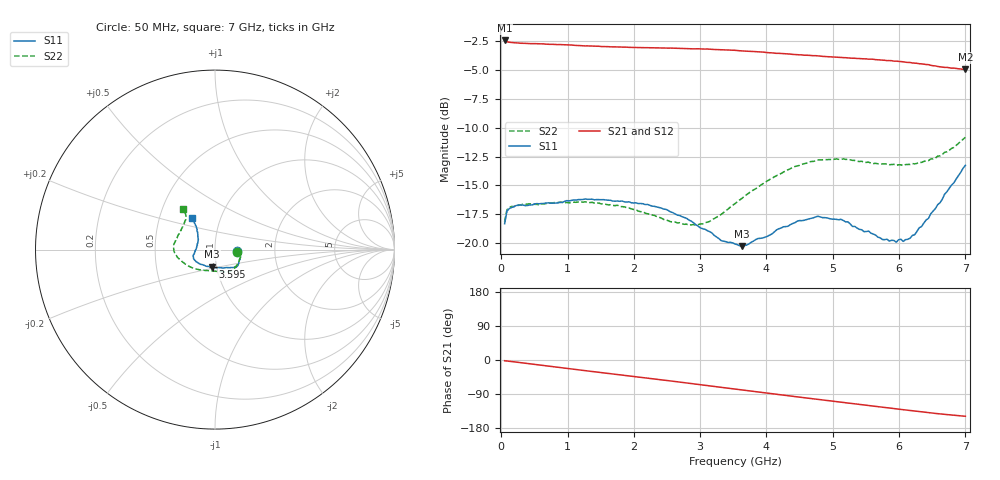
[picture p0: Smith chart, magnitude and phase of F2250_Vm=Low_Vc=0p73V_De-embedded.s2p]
! Integrated Device Technology
! Corporate Headquarters
! 6024 Silver Creek Valley Road
! San Jose, CA 95138  USA
! Phone:  1-408-284-8200
! Toll Free:  1-800-223-1366
! Webpage:  http://www.idt.com/
! Timing and RF Division
! 515 Groton Road, Suite 102
! Westford, MA 01886-6024
! Device:  F2250
! Description: Voltage Variable RF Attenuator
! Frequency:  50.0 -  6000.00 MHz
! Package:  3x3 mm Thin QFN Plastic Package: 16 pin
! Ports:  2 RF, 3 DC
!  Pin  1  = GND
!  Pin  2  = NC
!  Pin  3  = RF1  = Port 1
!  Pin  4  = NC
!  Pin  5  = GND
!  Pin  6  = GND
!  Pin  7  = GND
!  Pin  8  = GND
!  Pin  9  = NC
!  Pin 10  = RF2  = Port 2
!  Pin 11  = NC
!  Pin 12  = GND
!  Pin 13  = GND
!  Pin 14  = VCNTRL
!  Pin 15  = VDD
!  Pin 16  = VMODE
! Vcntrl:  0.730 Volts
! Vmode:  +0.000 Volts
! Vdd:  +3.30  Volts
! Current:  1.156 mA
! Data:  The device was measured on a the F2250 evaluation board which has
!  individual transmission lines to the RF pins.  Data was collected
!  using a calibrated network analyzer.  The evaluation board was
!  de-embedded using a TRL calibration technique.
!  The reference plane is the edge of the package pin.
! Misc:  SN 10
!  Action Tracker AT0258
! Date Measured:  2014-11-26
! Date:  2015-10-15  MJV
! Note:
!  Integrated Device Technology supplies this data as a sample of measured
!  data at the package pin for this product.  Your particular data for this
!  product may vary.
!  Data was taken at 25 degrees C.
!  Integrated Device Technology reserves the right to change this data at anytime.
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# GHz S dB R 50
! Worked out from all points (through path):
!   201 points, 50 MHz to 7 GHz, reference 50 ohm
!   highest |S21| = -2.45 dB at 50 MHz (marker M1); lowest = -5.0 dB at 7 GHz (marker M2)
!   group delay of S21, straight-line fit = 59.6 ps
!   lowest |S11| = -20.3 dB at 3.629 GHz (marker M3), VSWR 1.21, Z = 47.5 - j9.18 ohm
!   |S11| at or under -10 dB: start of sweep to end of sweep
!   |S22| runs from -18.4 to -10.8 dB; largest |S21 - S12| = 0.0014
!   S11 on the Smith chart (normalised r, x): 50 MHz: 1.28, -0.02; 3.595 GHz: 0.96, -0.19; 7 GHz: 0.73, +0.27
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0.05  -18.32 -4.1  -2.45 -2.0  -2.44 -2.0  -18.16 -5.6
0.08475  -17.23 -4.1  -2.57 -2.6  -2.56 -2.6  -17.11 -5.3
0.22375  -16.74 -7.7  -2.66 -5.5  -2.66 -5.5  -16.77 -10.0
0.64075  -16.56 -19.7  -2.75 -14.7  -2.76 -14.7  -16.60 -25.7
1.2315  -16.22 -34.0  -2.91 -27.4  -2.91 -27.4  -16.44 -46.5
1.75275  -16.35 -40.4  -3.01 -38.3  -3.01 -38.3  -16.71 -58.4
2.37825  -16.91 -44.3  -3.10 -51.5  -3.10 -51.5  -17.76 -72.1
2.93425  -18.40 -56.1  -3.17 -63.6  -3.17 -63.6  -18.45 -97.1
3.14275  -19.00 -66.3  -3.21 -68.2  -3.22 -68.2  -18.12 -110.4
3.3165  -19.78 -76.9  -3.26 -72.1  -3.25 -72.1  -17.51 -120.9
3.525  -20.07 -92.1  -3.30 -76.7  -3.31 -76.7  -16.58 -132.6
3.5945  -20.23 -97.0  -3.34 -78.3  -3.34 -78.3  -16.26 -135.9
3.62925  -20.26 -99.7  -3.36 -79.0  -3.35 -79.1  -16.13 -137.6
4.2895  -18.57 -139.1  -3.61 -93.5  -3.60 -93.5  -13.74 -165.1
4.7065  -17.81 -154.3  -3.77 -102.5  -3.76 -102.5  -12.92 -176.1
5.1235  -17.93 -164.2  -3.92 -111.3  -3.92 -111.4  -12.74 174.3
5.85325  -19.82 171.1  -4.19 -126.7  -4.19 -126.7  -13.21 156.6
6.027  -19.66 161.3  -4.28 -130.4  -4.28 -130.4  -13.22 151.3
6.06175  -19.85 160.0  -4.30 -131.1  -4.31 -131.1  -13.29 150.4
6.2355  -19.27 148.2  -4.42 -134.8  -4.42 -134.8  -13.14 144.4
6.61775  -16.50 131.5  -4.73 -142.2  -4.73 -142.2  -12.44 132.3
7  -13.26 126.4  -4.96 -148.4  -4.97 -148.5  -10.83 128.0
